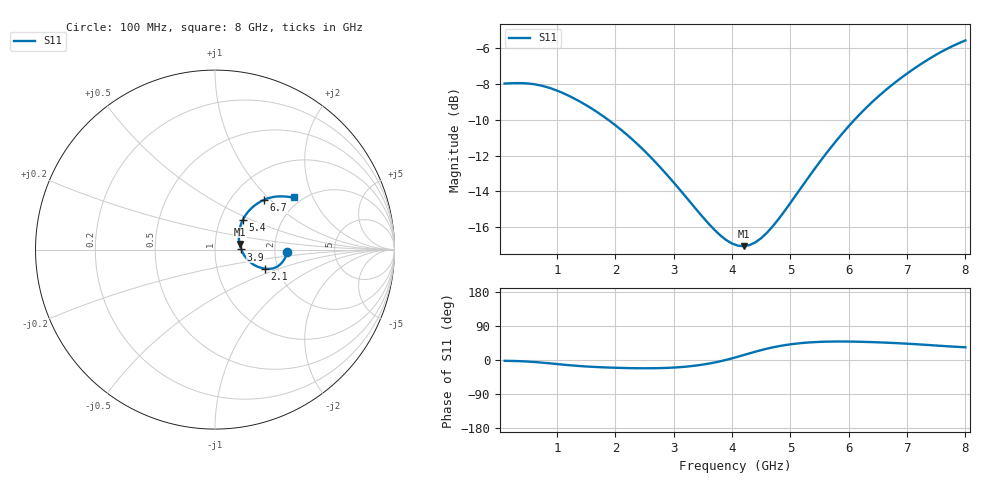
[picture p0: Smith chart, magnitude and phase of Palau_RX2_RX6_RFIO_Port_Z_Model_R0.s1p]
! Created Fri Jul 17 10:52:16 2020
! Palau RX2/RX6 RFIO Port Impedance Model.
! Revision		: R0.
! Impedance Mode 	: Balanced Differential-Mode.
! Impedance Format 	: Series Equivalent Differential Impedance (SEDZ).
# hz S ma R 50
! 1 Port Network Data from SP1.SP block
! freq  magS11  angS11
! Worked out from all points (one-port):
!   80 points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, 100 MHz to 8 GHz, reference 50 ohm
!   lowest |S11| = -17.0 dB at 4.2 GHz (marker M1), VSWR 1.33, Z = 65.7 + j4.28 ohm
!   |S11| at or under -10 dB: 1.872 GHz to 6.101 GHz (4.229 GHz wide, 106 % of centre)
!   S11 on the Smith chart (normalised r, x): 100 MHz: 2.32, -0.08; 2.1 GHz: 1.71, -0.40; 3.9 GHz: 1.34, +0.00; 5.4 GHz: 1.28, +0.45; 6.7 GHz: 1.40, +0.92; 8 GHz: 1.81, +1.45
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1e8  0.3987 -2.1
4e8  0.3997 -3.4
6e8  0.3971 -5.2
8e8  0.3906 -7.7
1.1e9  0.375 -12.2
1.3e9  0.3617 -14.9
1.6e9  0.339 -18.0
2.1e9  0.2961 -20.9
2.6e9  0.2491 -21.8
3.1e9  0.2022 -18.9
3.6e9  0.1622 -9.6
3.8e9  0.1505 -3.3
3.9e9  0.1461 0.4
4.1e9  0.141 8.7
4.2e9  0.1405 13.1
4.3e9  0.1415 17.6
4.4e9  0.144 21.9
4.6e9  0.1533 29.9
4.8e9  0.1675 36.5
5.1e9  0.1955 43.3
5.4e9  0.2289 47.1
5.8e9  0.2779 48.8
6.1e9  0.3161 48.4
6.4e9  0.3538 47.2
6.7e9  0.3902 45.3
7.1e9  0.4363 42.2
7.6e9  0.4898 37.1
8e9  0.5254 33.6
